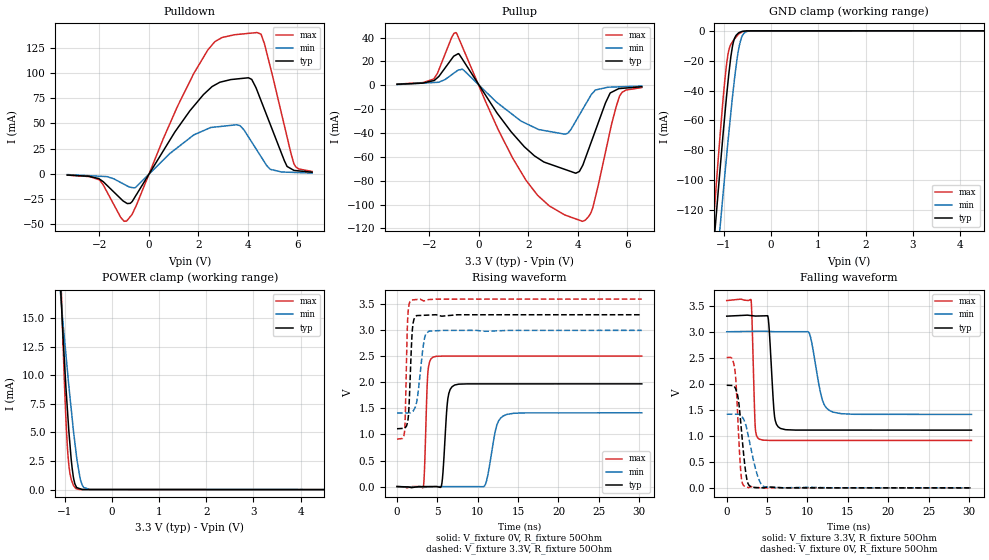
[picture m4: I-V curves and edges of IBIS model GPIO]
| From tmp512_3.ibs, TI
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|   GPIO   3.3V digital I/O_open_drain
[Model] GPIO
Model_type I/O
Polarity   Non-Inverting
Enable   Active-Low
Vinl = 0.8
Vinh = 2.1
Vmeas = 1.55
Vref = 1.55
Cref = 15pF
Rref = 50
|   typ   min   max
|   high inpedance in
C_comp   2.3008890e-12   1.8563280e-12   2.7705950e-12
|   output high
|C_comp   5.3278220e-12   3.9666320e-12   9.7896140e-12
|   output low
|C_comp   3.7165690e-12   3.6839090e-12   4.9230260e-12
[Voltage Range]   3.3   3   3.6
[Temperature Range]   27   125   -40
[GND Clamp Reference]   0   0   0
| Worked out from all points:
|   slope of the pulldown table from 0 to 0.495 V, typ, clamps not added: 25 ohm
|   slope of the pullup table from 0 to 0.495 V, typ, clamps not added: 31 ohm
|   GND clamp passes 1 mA (typ) near -0.67 V on its own axis
|   POWER clamp passes 1 mA (typ) near -0.81 V on its own axis
|   falling waveform, V_fixture 3.3V, R_fixture 50Ohm: 20-80 % time 486ps typ, 1.12ns min, 294ps max; typ from 3.3 V to 1.11 V
|   rising waveform, V_fixture 0V, R_fixture 50Ohm: 20-80 % time 474ps typ, 961ps min, 306ps max; typ from 0 V to 1.97 V
|   rising waveform, V_fixture 3.3V, R_fixture 50Ohm: 20-80 % time 349ps typ, 692ps min, 243ps max; typ from 1.11 V to 3.3 V
|   falling waveform, V_fixture 0V, R_fixture 50Ohm: 20-80 % time 733ps typ, 1.23ns min, 497ps max; typ from 1.97 V to 0 V
[Pulldown]
|   Voltage   I(typ)   I(min)   I(max)
-3.3V     -1.194mA   -714.8uA   -1.255mA
-2.004V   -5.101mA   -2.351mA   -5.945mA
-906.3mV  -28.95mA   -11.63mA   -46.71mA
-534.5mV  -21.62mA   -13.25mA   -32.37mA
1.147V    44.96mA    25.92mA    66.54mA
2.368V    82.28mA    44.57mA    122.3mA
3.682V    94.28mA    47.68mA    138.2mA
4.36V     83.03mA    23.46mA    139.9mA
4.66V     64.07mA    11.9mA     129.2mA
5.579V    7.356mA    1.669mA    36.53mA
5.85V     3.542mA    1.431mA    10.29mA
6.59V     1.624mA    782.7uA    2.368mA
[GND Clamp]
|   Voltage   I(typ)   I(min)   I(max)
-3.3V     -996.9mA   -969.2mA   -1.072A
-1.224V   -146.9mA   -182.1mA   -129.2mA
-1.184V   -131.1mA   -167.6mA   -112.1mA
-1.079V   -91.36mA   -130.2mA   -68.69mA
-986mV    -58.01mA   -98.05mA   -34.62mA
-939.8mV  -42.29mA   -82.65mA   -21.23mA
-882.8mV  -25.09mA   -64.04mA   -11.37mA
-815.9mV  -9.837mA   -43.37mA   -7.143mA
-679.6mV  -1.173mA   -10.78mA   -1.959mA
-586.6mV  -270.9uA   -2.047mA   -457.9uA
-408.5mV  -29.93uA   -25uA      -55.85uA
6.59V     0A         0A         0A
[Pullup]
|   Voltage   I(typ)   I(min)   I(max)
-3.3V     846.3uA    592.4uA    966.4uA
-1.815V   3.917mA    2.297mA    5.306mA
-922.9mV  25.39mA    11.36mA    44.2mA
-619.6mV  20.58mA    12.94mA    30.3mA
783.7mV   -24.45mA   -15.18mA   -36.98mA
1.896V    -52.53mA   -31.89mA   -79.17mA
3.499V    -70.68mA   -41.04mA   -108.9mA
4.189V    -67.7mA    -20.61mA   -114.1mA
4.609V    -44.1mA    -6.405mA   -102.7mA
5.308V    -6.625mA   -1.556mA   -38.37mA
5.691V    -2.743mA   -1.287mA   -9.111mA
6.59V     -1.212mA   -656.8uA   -1.876mA
[POWER Clamp]
|   Voltage   I(typ)   I(min)   I(max)
-3.3V     254.6mA    177.9mA    365.8mA
-1.084V   17.76mA    17.12mA    19.56mA
-1.051V   15.04mA    15.5mA     15.2mA
-986mV    10.05mA    12.5mA     7.644mA
-958.4mV  8.196mA    11.27mA    5.121mA
-922.9mV  6.002mA    9.695mA    2.786mA
-882.8mV  3.846mA    8.028mA    1.364mA
-838.9mV  1.883mA    6.254mA    672.6uA
-757.6mV  297.4uA    3.312mA    88uA
-627.9mV  13.62uA    418.3uA    8.843uA
-460.7mV  4.963uA    4.797uA    8.639uA
6.59V     0A         0A         0A
[Ramp]
R_load = 50
|   typ   min   max
dV/dt_r   1.18358/4.68423e-010  0.849656/9.48975e-010   1.50375/3.05611e-010
dV/dt_f   1.31417/4.83194e-010  0.953152/1.10861e-009   1.6132/2.9135e-010
[Falling Waveform]
V_fixture = 3.3V
V_fixture_min = 3V
V_fixture_max = 3.6V
R_fixture = 50Ohm
C_fixture = 0F
|   Time   V(typ)   V(min)   V(max)
0s        3.3V       3V         3.6V
3.009ns   3.312V     3.008V     3.616V
3.523ns   3.303V     3.009V     1.191V
4.018ns   3.304V     3.011V     936.4mV
5.11ns    3.289V     3.007V     913.4mV
5.904ns   1.398V     3.002V     911.7mV
6.659ns   1.142V     3.001V     911.7mV
10.19ns   1.11V      2.984V     911.7mV
13.16ns   1.11V      1.456V     911.6mV
30.32ns   1.11V      1.411V     911.3mV
[Rising Waveform]
V_fixture = 0V
V_fixture_min = 0V
V_fixture_max = 0V
R_fixture = 50Ohm
C_fixture = 0F
|   Time   V(typ)   V(min)   V(max)
0s        558.5pV    965.3pV    485.1pV
3.253ns   -526.8uV   -14.66mV   -13.77mV
3.809ns   -251.8uV   -10.78mV   2.164V
4.439ns   59.21uV    -3.691mV   2.485V
5.497ns   12.04mV    -805.2uV   2.505V
6.286ns   1.678V     -995.9uV   2.506V
7.122ns   1.949V     -1.198mV   2.506V
10.86ns   1.972V     15.31mV    2.506V
13.58ns   1.972V     1.385V     2.506V
30.32ns   1.973V     1.416V     2.506V
[Rising Waveform]
V_fixture = 3.3V
V_fixture_min = 3V
V_fixture_max = 3.6V
R_fixture = 50Ohm
C_fixture = 0F
|   Time   V(typ)   V(min)   V(max)
0s        1.11V      1.411V     911.3mV
931.2ps   1.12V      1.413V     1.058V
1.326ns   1.247V     1.414V     3.24V
1.485ns   1.54V      1.415V     3.496V
1.769ns   2.64V      1.426V     3.582V
1.988ns   3.135V     1.449V     3.586V
2.232ns   3.258V     1.513V     3.59V
3.366ns   3.29V      2.818V     3.566V
3.955ns   3.294V     2.984V     3.592V
30.32ns   3.3V       3V         3.6V
[Falling Waveform]
|Gnd
V_fixture = 0V
V_fixture_min = 0V
V_fixture_max = 0V
R_fixture = 50Ohm
C_fixture = 0F
|   Time   V(typ)   V(min)   V(max)
0s        1.973V     1.416V     2.506V
1.002ns   1.933V     1.415V     2.278V
1.169ns   1.874V     1.415V     1.974V
1.44ns    1.701V     1.415V     1.123V
1.755ns   1.222V     1.393V     281.8mV
2.266ns   401.4mV    1.256V     20.89mV
2.776ns   45.64mV    919.7mV    8.64mV
3.786ns   4.463mV    247.1mV    4.612mV
4.698ns   4.734mV    18.83mV    279.8uV
30.32ns   199.2nV    382.8nV    119.9nV
